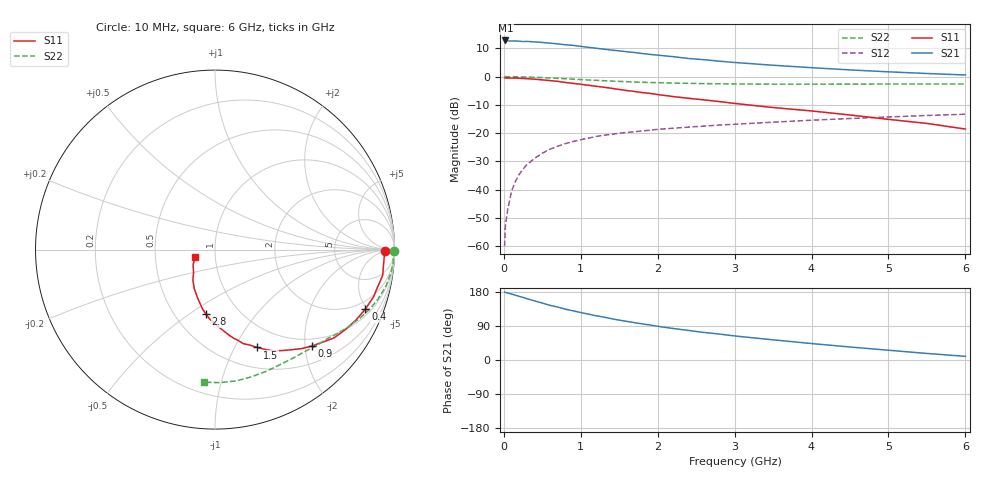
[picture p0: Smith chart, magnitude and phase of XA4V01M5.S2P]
! SIEMENS Discrete & RF Semiconductors
! BFY180
! Si NPN RF Bipolar Junction Transistor in MICRO-X
! VCE = 4 V  IC = 1.5 mA
! Common Emitter S-Parameters:  May  1997
# GHz  S  MA  R  50
!  f  S11  S21  S12  S22
! GHz  MAG  ANG  MAG  ANG  MAG  ANG  MAG  ANG
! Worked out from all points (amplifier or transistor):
!   36 points, 10 MHz to 6 GHz, reference 50 ohm
!   highest |S21| = 12.8 dB at 20 MHz (marker M1)
!   |S21| within 3 dB of that: start of sweep to 1.274 GHz
!   unconditionally stable (mu >= 1): 3.305 GHz to end of sweep
!   at 250 MHz: K = 0.10, MSG = 22.6 dB, |S12| = -32.7 dB
!   at 1.4 GHz: K = 0.59, MSG = 14.9 dB, |S12| = -20.4 dB
!   at 6 GHz: K = 1.07, MAG = 5.4 dB, |S12| = -13.3 dB
!   S11 on the Smith chart (normalised r, x): 10 MHz: 37, -6; 400 MHz: 1.38, -4.87; 900 MHz: 0.84, -2.14; 1.5 GHz: 0.73, -1.23; 2.8 GHz: 0.70, -0.58; 6 GHz: 0.80, -0.07
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0.01  0.9481 -0.5  4.279 179.2  0.001 94.5  0.9959 -0.3
0.02  0.9464 -1.1  4.37 178.4  0.0023 88.5  0.9989 -0.6
0.05  0.9437 -2.6  4.285 177.0  0.0044 85.9  0.9969 -1.5
0.1  0.9428 -5.6  4.269 174.1  0.0094 87.2  0.9942 -3.0
0.15  0.9454 -8.6  4.282 171.0  0.0139 85.9  0.9953 -4.6
0.25  0.9274 -13.7  4.177 165.2  0.0231 81.4  0.9889 -7.6
0.3  0.9223 -16.5  4.201 161.8  0.0277 79.4  0.9833 -8.9
0.4  0.9011 -21.6  4.127 156.0  0.0359 76.1  0.9749 -11.8
0.6  0.8507 -31.8  3.916 144.2  0.0521 69.6  0.9483 -17.0
0.8  0.7894 -40.9  3.669 134.2  0.0652 63.6  0.9181 -21.7
0.9  0.7608 -45.0  3.573 129.7  0.0712 60.9  0.9019 -24.0
1.1  0.7032 -52.5  3.299 121.0  0.0816 56.4  0.8722 -27.9
1.2  0.6753 -56.4  3.185 116.7  0.0874 54.3  0.8606 -29.8
1.5  0.5933 -66.7  2.862 105.2  0.0995 49.4  0.8235 -34.8
1.8  0.5222 -75.7  2.565 95.3  0.1097 45.7  0.7949 -39.3
2.2  0.4438 -85.5  2.258 83.2  0.1223 41.3  0.7711 -44.9
2.6  0.388 -94.4  1.997 72.7  0.1333 37.8  0.7534 -50.0
2.8  0.3622 -98.1  1.878 68.5  0.1392 36.4  0.7481 -52.5
3.5  0.2841 -110.2  1.591 53.2  0.1564 31.3  0.7362 -61.1
4.5  0.2095 -126.1  1.315 34.3  0.1818 24.1  0.7372 -74.0
5.5  0.1485 -145.2  1.137 17.3  0.2055 16.6  0.7418 -87.8
6  0.1183 -159.6  1.07 9.6  0.2165 12.3  0.7412 -94.8
